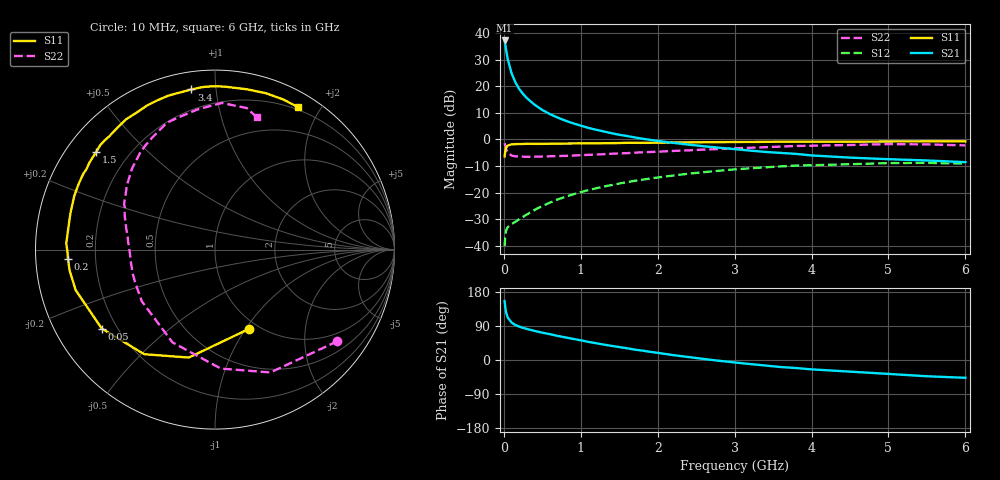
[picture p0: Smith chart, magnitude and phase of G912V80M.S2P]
! SIEMENS Small Signal Semiconductors
! BFG235
! Si NPN RF Bipolar Junction Transistor in SOT223
! VCE = 12 V  IC = 80 mA
! Common Emitter S-Parameters:  July  1994
# GHz  S  MA  R  50
!  f  S11  S21  S12  S22
! GHz  MAG  ANG  MAG  ANG  MAG  ANG  MAG  ANG
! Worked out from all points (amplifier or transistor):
!   40 points, 10 MHz to 6 GHz, reference 50 ohm
!   highest |S21| = 37.2 dB at 10 MHz (marker M1)
!   |S21| within 3 dB of that: start of sweep to 26.75 MHz
!   unconditionally stable (mu >= 1): 486.4 MHz to 1.438 GHz
!   at 200 MHz: K = 0.72, MSG = 24.4 dB, |S12| = -29.9 dB
!   at 1.5 GHz: K = 0.99, MSG = 9.2 dB, |S12| = -16.6 dB
!   at 6 GHz: K = 0.91, MSG = 0.3 dB, |S12| = -9.1 dB
!   S11 on the Smith chart (normalised r, x): 10 MHz: 0.90, -1.03; 50 MHz: 0.14, -0.31; 200 MHz: 0.10, -0.03; 1.5 GHz: 0.09, +0.36; 3.4 GHz: 0.09, +0.86; 6 GHz: 0.17, +1.73
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0.01  0.4809 -67.1  72.42 155.5  0.0099 65.8  0.8522 -36.8
0.02  0.6189 -103.6  59.2 137.7  0.0161 51.6  0.7509 -65.7
0.03  0.7038 -124.1  47.84 125.8  0.0196 43.1  0.6637 -87.2
0.05  0.7691 -145.1  32.71 112.2  0.0226 33.7  0.5685 -114.7
0.1  0.8085 -163.8  17.56 98.9  0.0258 33.3  0.4994 -144.7
0.15  0.8183 -171.8  11.84 92.3  0.0283 37.3  0.4814 -157.4
0.2  0.8206 -176.2  8.87 88.2  0.0319 41.6  0.4776 -164.3
0.25  0.8228 -179.7  7.146 84.8  0.0352 45.8  0.4741 -168.9
0.3  0.8295 177.7  5.971 82.0  0.039 49.0  0.4739 -172.5
0.4  0.8259 172.7  4.486 76.7  0.0475 53.3  0.4744 -177.2
0.5  0.8272 169.0  3.584 72.1  0.0563 55.8  0.4784 179.2
0.6  0.8307 165.7  2.988 68.1  0.0652 57.0  0.4832 176.2
0.7  0.8339 162.1  2.576 63.5  0.0748 57.7  0.4885 173.5
0.9  0.8409 156.6  2.013 55.7  0.0932 56.9  0.4992 169.1
1.1  0.8468 150.1  1.648 47.8  0.1118 55.1  0.5144 164.8
1.5  0.8567 140.5  1.225 34.1  0.1487 49.9  0.5468 156.9
2.2  0.8789 124.2  0.864 12.9  0.2101 38.0  0.6092 143.5
3.2  0.8967 102.8  0.618 -10.7  0.2874 18.7  0.6982 123.7
3.4  0.9018 98.4  0.583 -14.6  0.2996 14.6  0.7156 119.2
4.5  0.9108 78.7  0.456 -30.7  0.3431 -7.0  0.7875 96.9
5.5  0.9189 65.5  0.403 -42.9  0.3632 -25.7  0.8083 77.4
6  0.9188 59.6  0.375 -47.0  0.3521 -32.4  0.7744 72.6
